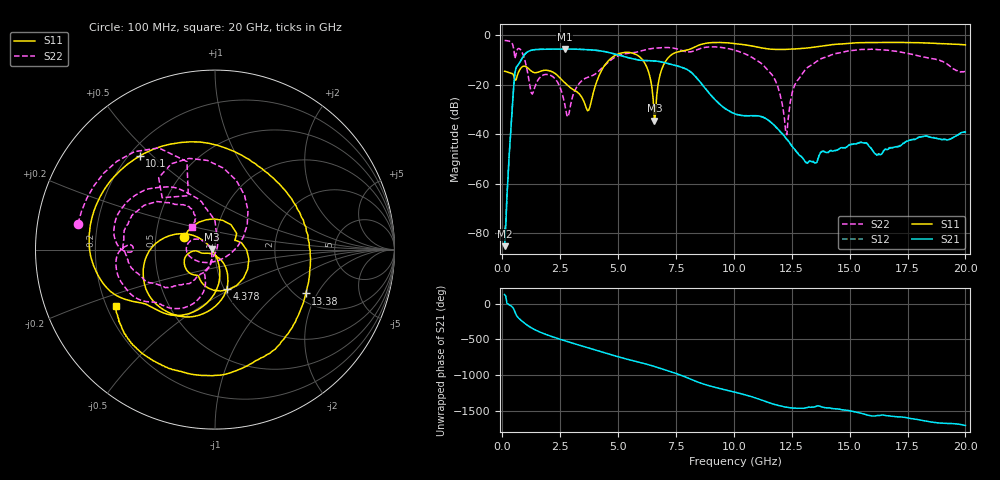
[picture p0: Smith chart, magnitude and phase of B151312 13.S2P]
!  2-Port S-parameters saved by WinCal
! VAR MeasName=S-Parameters (CALIBRATED_DATA) read from VNA (N5244A)
! VAR MeasDate=12/8/2015 5:44:35 PM
! VAR NAME=B151312 13
! VAR FILENAME=B151312 13.S2P
! VAR DATE=12/8/2015 5:44:35 PM
! VAR PHYS_PORTS=1,2
# Hz S DB R 50
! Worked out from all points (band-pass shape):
!   401 points, 100 MHz to 20 GHz, reference 50 ohm
!   highest |S21| = -5.65 dB at 2.687 GHz (marker M1); lowest = -85.3 dB at 100 MHz (marker M2)
!   |S21| within 3 dB of the highest: 905.2 MHz to 5.239 GHz (4.333 GHz wide, 141 % of centre)
!   lowest |S11| = -34.6 dB at 6.567 GHz (marker M3), VSWR 1.04, Z = 48.2 + j0.339 ohm
!   |S11| at or under -10 dB: start of sweep to 4.629 GHz; 6.056 GHz to 7.097 GHz (1.041 GHz wide, 15.8 % of centre)
!   |S22| runs from -40.3 to -2.2 dB; largest |S21 - S12| = 0.0015
!   S11 on the Smith chart (normalised r, x): 100 MHz: 0.70, +0.10; 4.378 GHz: 1.03, -0.47; 10.1 GHz: 0.24, +0.46; 13.38 GHz: 2.25, -1.61; 20 GHz: 0.24, -0.25
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1e8  -14.65 157.5  -85.29 126.6  -79.08 124.5  -2.19 169.3
4.4825e8  -15.66 57.1  -26.94 -52.8  -26.95 -52.8  -3.77 118.9
6.4725e8  -16.35 14.6  -12.49 178.9  -12.49 178.9  -5.86 128.1
1.04525e9  -12.91 -92.3  -7.11 66.2  -7.11 66.2  -12.89 37.7
1.44325e9  -15.22 -123.4  -5.86 -10.4  -5.86 -10.4  -20.05 -134.8
2.13975e9  -14.80 -160.1  -5.71 -99.5  -5.71 -99.5  -16.61 162.4
2.687e9  -19.15 -176.5  -5.65 -157.1  -5.66 -157.1  -27.48 146.1
3.43325e9  -25.11 -158.0  -5.81 129.2  -5.81 129.2  -18.46 -113.3
3.73175e9  -30.35 -102.1  -5.92 100.2  -5.92 100.2  -16.96 -114.6
4.3785e9  -12.83 -73.4  -6.62 36.9  -6.62 36.9  -12.66 -105.1
5.871e9  -8.38 -175.1  -10.09 -95.3  -10.08 -95.5  -6.75 -140.6
6.5675e9  -34.57 169.2  -10.46 -156.9  -10.45 -157.0  -5.35 -155.9
6.7665e9  -17.94 -77.8  -10.68 -177.4  -10.68 -177.3  -5.14 -160.9
8.3585e9  -4.62 -152.8  -16.94 -4.2  -16.92 -4.6  -6.12 -178.7
1.005e10  -3.44 131.2  -31.83 -156.6  -31.87 -156.9  -6.14 136.3
1.009975e10  -3.49 128.8  -32.01 -160.3  -32.03 -160.6  -6.28 134.9
1.169175e10  -5.78 53.1  -35.95 38.6  -36.01 38.9  -16.61 89.4
1.2239e10  -5.82 25.8  -41.52 -4.1  -41.58 -3.4  -39.17 14.0
1.2637e10  -5.65 6.7  -46.22 -19.8  -46.32 -19.4  -20.02 -109.3
1.338325e10  -5.01 -25.8  -51.14 -4.5  -51.28 -4.2  -11.92 -130.3
1.67165e10  -3.00 -113.7  -45.74 -127.3  -45.49 -127.7  -6.21 154.8
2e10  -3.96 -150.4  -39.20 99.5  -39.19 98.2  -14.78 135.8
